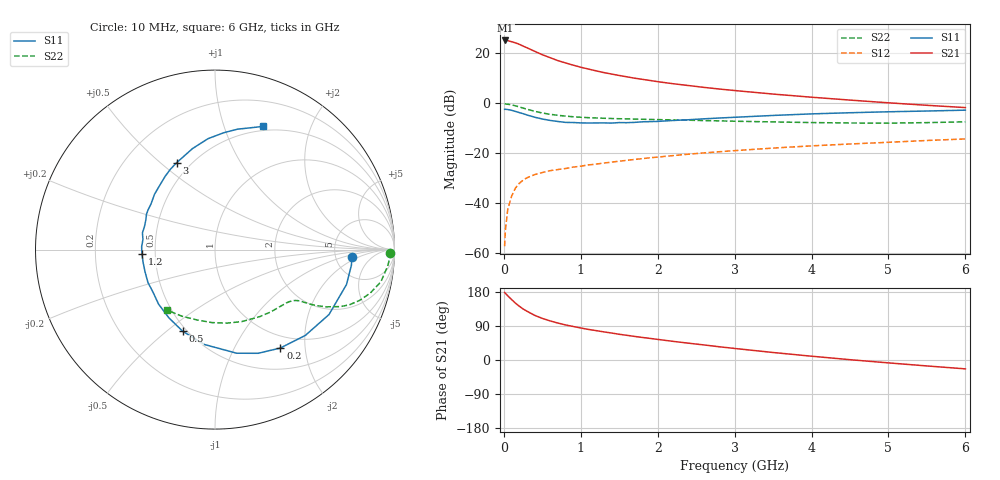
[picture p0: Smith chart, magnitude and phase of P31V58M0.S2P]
! SIEMENS Small Signal Semiconductors
! BFP181
! Si NPN RF Bipolar Junction Transistor in SOT143
! VCE = 1.5 V  IC = 8 mA
! Common Emitter S-Parameters:  March  1996
# GHz  S  MA  R  50
!  f  S11  S21  S12  S22
! GHz  MAG  ANG  MAG  ANG  MAG  ANG  MAG  ANG
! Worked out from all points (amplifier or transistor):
!   36 points, 10 MHz to 6 GHz, reference 50 ohm
!   highest |S21| = 25.2 dB at 20 MHz (marker M1)
!   |S21| within 3 dB of that: start of sweep to 305.7 MHz
!   unconditionally stable (mu >= 1): 1.049 GHz to end of sweep
!   at 250 MHz: K = 0.34, MSG = 26.8 dB, |S12| = -30.7 dB
!   at 1.4 GHz: K = 1.14, MAG = 15.3 dB, |S12| = -23.5 dB
!   at 6 GHz: K = 1.05, MAG = 4.9 dB, |S12| = -14.2 dB
!   S11 on the Smith chart (normalised r, x): 10 MHz: 7.16, -1.42; 200 MHz: 0.80, -1.56; 500 MHz: 0.48, -0.57; 1.2 GHz: 0.42, -0.02; 3 GHz: 0.42, +0.57; 6 GHz: 0.45, +1.36
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0.01  0.7633 -3.1  18.14 178.0  0.0014 79.3  0.9744 -1.0
0.02  0.765 -6.6  18.22 176.2  0.0029 80.5  0.9776 -2.2
0.05  0.758 -14.9  18.08 169.5  0.0075 87.1  0.9655 -5.7
0.1  0.7309 -29.7  17.2 159.7  0.0139 74.4  0.9412 -11.0
0.15  0.6943 -43.5  16.34 150.2  0.0202 67.9  0.8988 -15.6
0.2  0.6583 -56.4  15.29 142.0  0.0252 64.2  0.8549 -19.3
0.25  0.6258 -67.4  14.06 134.7  0.0293 59.7  0.8098 -22.3
0.3  0.5897 -78.2  13.02 128.8  0.0326 55.8  0.7687 -24.4
0.4  0.5321 -96.3  11.06 117.9  0.0378 51.1  0.6976 -27.2
0.5  0.4893 -111.6  9.446 109.8  0.0416 48.0  0.6457 -28.9
0.6  0.4587 -124.1  8.267 103.3  0.0453 46.6  0.6083 -29.9
0.7  0.4372 -136.0  7.225 97.6  0.0477 45.7  0.58 -30.5
0.9  0.4161 -153.9  5.848 88.5  0.0534 44.9  0.5428 -31.6
1.1  0.4069 -170.0  4.882 80.7  0.0591 45.3  0.5204 -33.1
1.2  0.408 -176.7  4.488 77.5  0.0613 44.5  0.5131 -34.0
1.7  0.4191 156.9  3.207 62.2  0.076 45.1  0.4876 -39.3
2.2  0.4571 137.4  2.485 49.2  0.0908 43.6  0.4693 -46.3
3  0.5293 113.8  1.816 30.5  0.114 39.6  0.4414 -59.7
3.5  0.5764 102.6  1.542 19.8  0.1282 36.5  0.4279 -69.6
4.5  0.653 85.7  1.169 0.8  0.1548 29.0  0.4071 -92.4
5.5  0.7066 73.8  0.92 -15.7  0.182 22.2  0.4142 -116.3
6  0.7353 68.9  0.828 -23.4  0.1953 18.2  0.4298 -128.2
